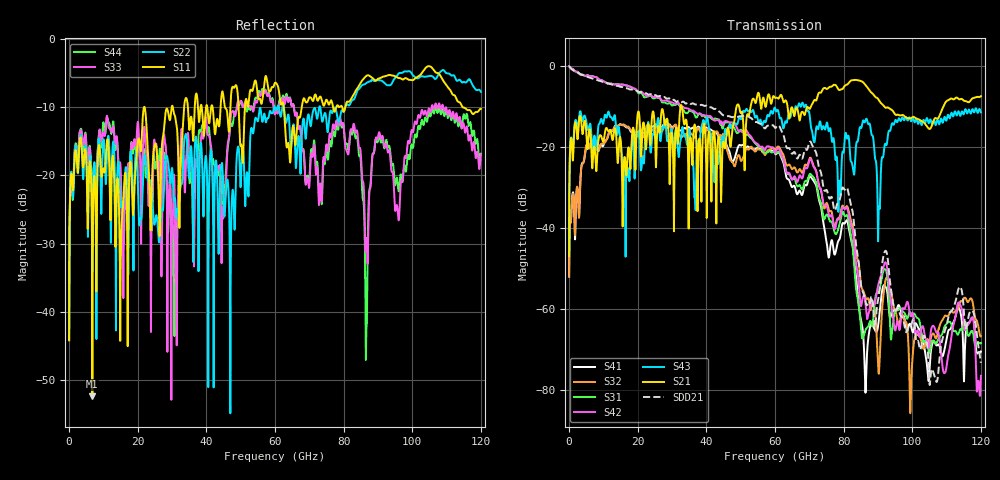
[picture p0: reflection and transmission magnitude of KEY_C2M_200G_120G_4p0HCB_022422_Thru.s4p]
! Touchstone file
!  Generated:  6:12:31 AM  Oct 19, 2021
!  Setup:  LinearFrequency
!  Solution:  LinearFrequency
# GHz S MA R 50.000000
! Terminal data exported
! Port[1] = P1
! Port[2] = P3
! Port[3] = P2
! Port[4] = P4
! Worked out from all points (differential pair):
!   12000 points, 10 MHz to 120 GHz, reference 50 ohm
!   strongest paths, dB at 10 MHz, 30.01 GHz, 60.01 GHz, 90.01 GHz, 120 GHz:
!     S21: -47.0, -17.0, -7.9, -8.1, -7.5
!     S43: -46.9, -16.1, -10.4, -42.2, -11.5
!     S42: -0.1, -9.0, -21.4, -54.4, -76.5
!     S31: -0.1, -9.8, -21.5, -56.1, -68.4
!     S32: -52.0, -15.8, -20.7, -73.7, -66.7
!     S41: -52.0, -15.1, -21.7, -64.4, -70.5
!   taken as a pair (ports 2,1 in; 4,3 out), SDD21 dB: -0.1, -8.5, -15.3, -57.9, -73.3
!   lowest |S11| = -52.4 dB at 6.78 GHz (marker M1), VSWR 1.00, Z = 50.1 - j0.217 ohm
!   |S11| at or under -10 dB: start of sweep to 21.81 GHz; 22.03 GHz to 29.89 GHz (7.862 GHz wide, 30.3 % of centre); 114.8 GHz to end of sweep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
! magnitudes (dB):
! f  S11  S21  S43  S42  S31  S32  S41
! 10 MHz  -44.2  -47.0  -46.9  -0.1  -0.1  -52.0  -52.0
! 6.78 GHz  -52.4  -25.2  -20.7  -2.5  -2.5  -18.6  -18.6
! 70.39 GHz  -8.6  -10.2  -14.5  -23.0  -26.7  -22.7  -27.3
! 81.29 GHz  -9.2  -4.4  -17.3  -36.0  -37.6  -35.2  -39.0
! 86.41 GHz  -5.5  -4.8  -13.4  -58.8  -65.1  -57.2  -80.3
! 90.26 GHz  -5.8  -8.4  -35.1  -53.5  -55.9  -75.9  -62.7
! 120 GHz  -10.2  -7.5  -11.5  -76.5  -68.4  -66.7  -70.5
